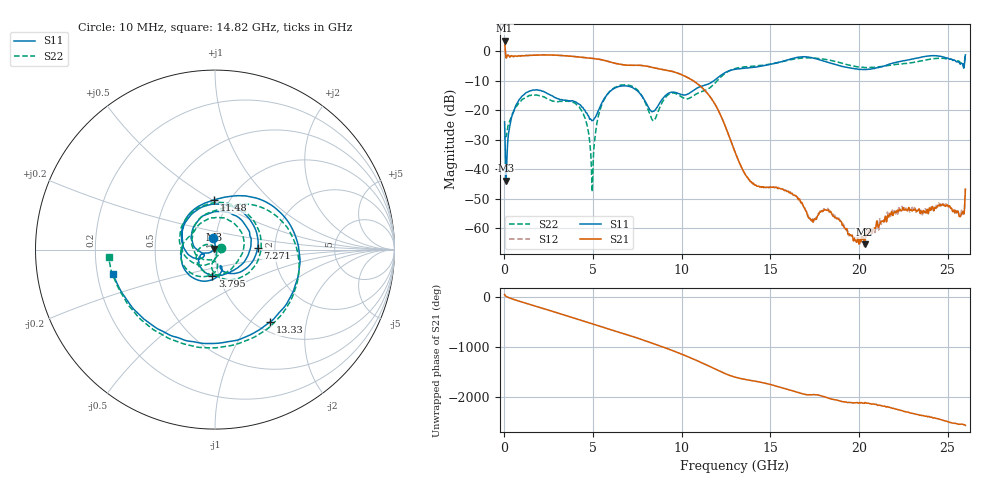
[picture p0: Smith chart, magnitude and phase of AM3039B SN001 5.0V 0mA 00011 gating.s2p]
!Agilent Technologies,E8364B,MY43040894,A.07.50.67
!Agilent E8364B: A.07.50.67
!Date: Tuesday, June 28, 2016 08:03:59
!Correction: S11(Full 2 Port(1,2))
!S21(Full 2 Port(1,2))
!S12(Full 2 Port(1,2))
!S22(Full 2 Port(1,2))
!S2P File: Measurements: S11, S21, S12, S22:
# Hz S  dB  R 50
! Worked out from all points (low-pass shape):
!   1601 points, 10 MHz to 26 GHz, reference 50 ohm
!   highest |S21| = 3.56 dB at 10 MHz (marker M1); lowest = -65.4 dB at 20.31 GHz (marker M2)
!   |S21| within 3 dB of the highest: start of sweep to 44.58 MHz
!   lowest |S11| = -43.8 dB at 91.22 MHz (marker M3), VSWR 1.01, Z = 49.5 + j0.354 ohm
!   |S11| at or under -10 dB: start of sweep to 11.82 GHz
!   |S22| runs from -47.6 to -0.8 dB; largest |S21 - S12| = 0.024
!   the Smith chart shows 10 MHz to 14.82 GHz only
!   S11 on the Smith chart (normalised r, x): 10 MHz: 0.97, +0.12; 3.795 GHz: 0.93, -0.28; 7.271 GHz: 1.62, +0.03; 11.48 GHz: 0.85, +0.51; 13.33 GHz: 1.16, -1.25; 14.82 GHz: 0.27, -0.11
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1e7  -23.93 98.8  3.56 40.4  3.61 41.3  -28.88 16.1
9.121875e7  -43.84 146.1  -2.22 4.9  -2.12 4.9  -28.88 -57.9
7.572125e8  -17.25 158.7  -1.66 -82.8  -1.61 -82.7  -18.02 173.8
1.634375e9  -13.12 68.6  -1.38 -177.4  -1.34 -177.3  -14.70 73.0
2.592756e9  -14.85 -16.9  -1.31 80.1  -1.27 80.2  -16.59 -15.2
3.794794e9  -16.75 -95.7  -1.74 -50.4  -1.72 -50.3  -17.10 -110.2
4.347081e9  -18.77 -141.0  -2.09 -111.2  -2.06 -111.0  -20.05 -171.0
4.9481e9  -23.50 -154.7  -2.47 -178.0  -2.42 -177.8  -47.59 32.4
5.695312e9  -15.52 -179.7  -3.24 96.6  -3.19 96.8  -15.65 -164.2
7.270956e9  -12.50 2.1  -4.80 -76.1  -4.77 -76.1  -12.10 -11.2
8.684162e9  -18.26 -72.0  -5.96 112.3  -5.91 112.2  -20.25 -81.5
1.147809e10  -11.18 91.4  -14.50 70.8  -14.48 70.4  -12.84 82.5
1.3005e10  -6.17 -25.7  -34.13 -157.5  -34.16 -158.1  -5.90 -32.9
1.332988e10  -5.90 -52.7  -38.76 173.8  -38.78 173.3  -5.50 -60.9
1.48243e10  -4.68 -166.3  -46.05 71.4  -46.03 71.3  -4.52 -175.9
1.622126e10  -2.54 80.5  -48.10 -66.2  -48.16 -66.4  -2.83 76.8
1.734208e10  -2.24 -26.4  -57.04 -147.2  -57.23 -143.4  -2.29 -18.3
2.031469e10  -6.22 102.6  -65.39 50.1  -65.08 54.9  -5.54 111.3
2.167916e10  -4.45 11.9  -56.13 -33.2  -55.27 -33.7  -4.86 17.1
2.416446e10  -1.53 179.0  -52.86 113.3  -53.07 120.7  -2.57 -166.8
2.513908e10  -2.68 95.6  -52.75 21.8  -52.79 23.8  -2.74 111.5
2.6e10  -1.26 -25.7  -46.70 -35.9  -46.71 -38.7  -0.81 1.5
